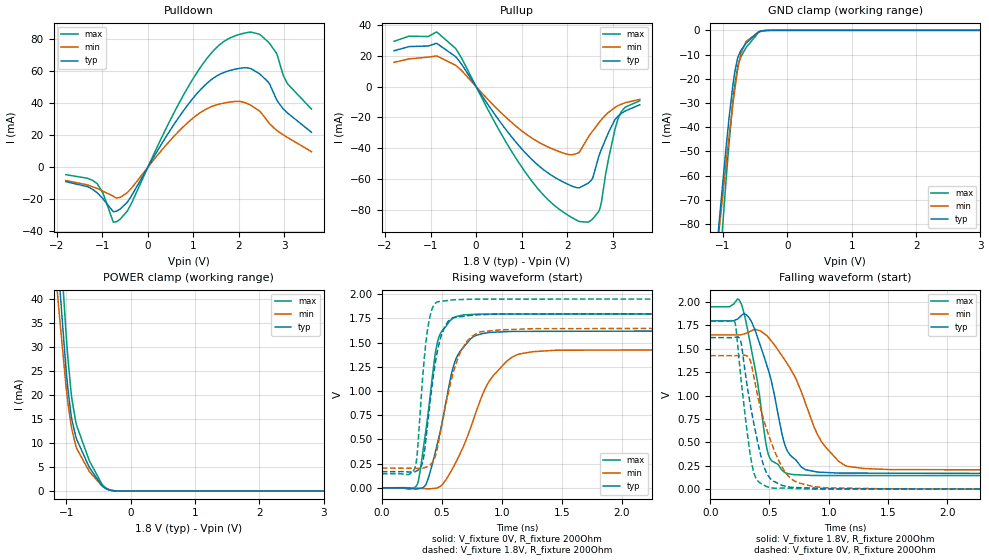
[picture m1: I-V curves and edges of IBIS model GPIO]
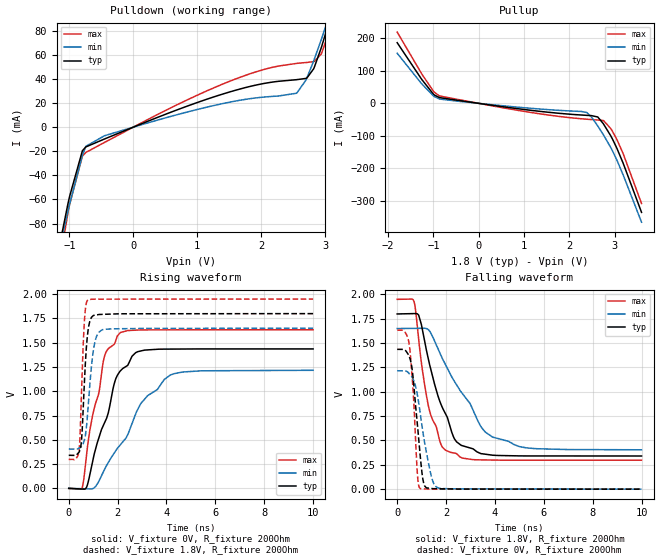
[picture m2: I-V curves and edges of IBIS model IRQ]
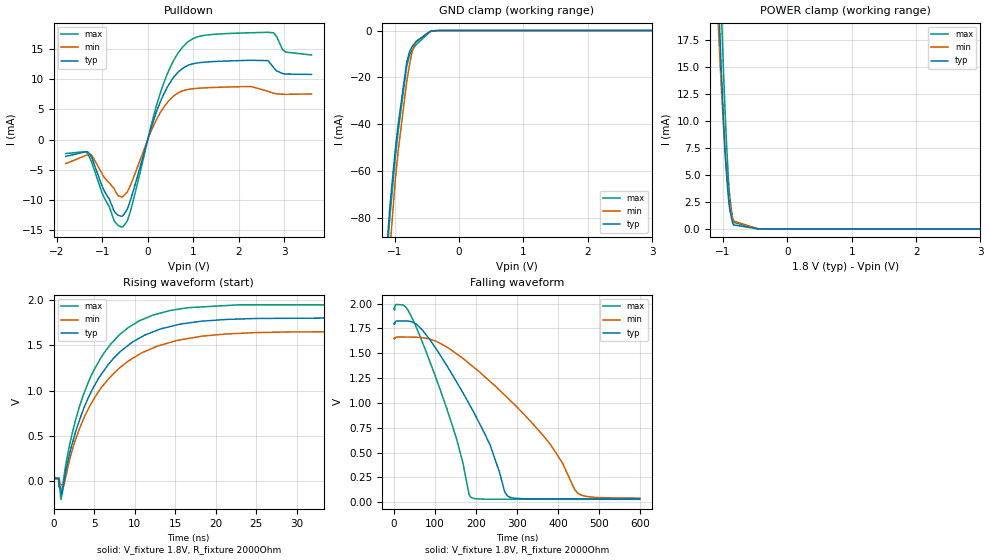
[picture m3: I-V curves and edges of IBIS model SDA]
|Texas Instruments Incorporated
| MIPI DSI Bridge To eDP
| Marketing part#   Digital Voltage Range   Package-type   #pins
| SN65DSI86   1.65V-1.95   PBGA   81
[IBIS Ver]   4.1
[File name]   sn65dsi86.ibs
[File Rev]   1.0
[Date]   09/19/2013
[Source]
| Texas Instruments Incorporated.
| Analog-eLab Design Center, HPA
| 12500 TI Blvd
| Dallas, TX -75243
| e-mail: elab_scm_ibis@list.ti.com
[Notes]   Revision History:
| Rev 1.0: 09/19/2013
| - Initial version of the model
| - Model generated from simulations in TISPICE
| - C_comp although listed in numerical order of value are
|   obtained from varying PVT conditions. For PVT conditions for
|   each specific value refer the buffer description under
|   respective [Model]. IBIS model user is responsible for using
|   appropriate C_comp to simulate for Signal Integrity.
| - Warnings regarding combined Non-monotonicity of various models have been
|   reviewd and considered minor and can be ignored.
| - DP output has sub models depending on the drive strength.
|   Please refer to the [Model Selector] section for details.
| - AUX pins has sub models depending on the drive strength.
|   Please refer to the [Model Selector] section for details.
[Disclaimer]
| This model is designed as an aid for customers of Texas Instruments.
| TI and its licensors and suppliers make no warranties, either expressed
| or implied, with respect to this  model, including the warranties of
| merchantability or fitness for a particular purpose. The model is
| provided solely on an "as is" basis. The entire risk as to its quality
| and performance is with the customer.
[Copyright]
 (C) Copyright 2013 Texas Instruments Incorporated.All rights reserved.
|   SN65DSI86
[Component]   SN65DSI86
[Manufacturer]   TI
[Package]
| variable   typ   min   max
R_pkg   0.1   0.08   0.12
L_pkg   0.7nH   0.56nH   0.84nH
C_pkg   0.1pF   0.08pF   0.12pF
[Pin]  signal_name   model_name   R_pin   L_pin   C_pin
A1   ADDR   input   NA   NA   NA
A2   VCCIO   POWER   NA   NA   NA
A3   IRQ   IRQ   NA   NA   NA
A4   GPIO1   GPIO   NA   NA   NA
A5   GPIO2   GPIO   NA   NA   NA
A6   GPIO3   GPIO   NA   NA   NA
A7   REFCLK   refclk_in   NA   NA   NA
A8   GND   GND   NA   NA   NA
A9   VCCA   POWER   NA   NA   NA
B1   EN   input_b   NA   NA   NA
B2   VCCA   POWER   NA   NA   NA
B3   TEST1   input_w_pd   NA   NA   NA
B4   GPIO4   GPIO   NA   NA   NA
B5   TEST2   input_w_pd   NA   NA   NA
B6   VCCIO   POWER   NA   NA   NA
B7   TEST3   input_w_pd   NA   NA   NA
B8   ML3P   DP_OUT   NA   NA   NA
B9   ML3N   DP_OUT   NA   NA   NA
C1   DB0N   DSI_INPUT   NA   NA   NA
C2   DB0P   DSI_INPUT   NA   NA   NA
C8   ML2P   DP_OUT   NA   NA   NA
C9   ML2N   DP_OUT   NA   NA   NA
D1   DB1N   DSI_INPUT   NA   NA   NA
D2   DB1P   DSI_INPUT   NA   NA   NA
D5   VCC   POWER   NA   NA   NA
D6   VCC   POWER   NA   NA   NA
D8   GND   GND   NA   NA   NA
D9   VPLL   POWER   NA   NA   NA
E1   DBCN   DSI_INPUT   NA   NA   NA
E2   DBCP   DSI_INPUT   NA   NA   NA
E4   GND   GND   NA   NA   NA
E5   GND   GND   NA   NA   NA
E6   VCCA   POWER   NA   NA   NA
E8   ML1P   DP_OUT   NA   NA   NA
E9   ML1N   DP_OUT   NA   NA   NA
F1   DB2N   DSI_INPUT   NA   NA   NA
F2   DB2P   DSI_INPUT   NA   NA   NA
F4   GND   GND   NA   NA   NA
F5   GND   GND   NA   NA   NA
F6   GND   GND   NA   NA   NA
F8   ML0P   DP_OUT   NA   NA   NA
F9   ML0N   DP_OUT   NA   NA   NA
G1   DB3N   DSI_INPUT   NA   NA   NA
G2   DB3P   DSI_INPUT   NA   NA   NA
G8   GND   GND   NA   NA   NA
G9   VCCA   POWER   NA   NA   NA
H1   SCL   SDA   NA   NA   NA
H2   VCCA   POWER   NA   NA   NA
H3   DA0P   LP_TX   NA   NA   NA
H4   DA1P   DSI_INPUT   NA   NA   NA
H5   DACP   DSI_INPUT   NA   NA   NA
H6   DA2P   DSI_INPUT   NA   NA   NA
H7   DA3P   DSI_INPUT   NA   NA   NA
H8   AUXP   AUX   NA   NA   NA
H9   AUXN   AUX   NA   NA   NA
J1   SDA   SDA   NA   NA   NA
J2   VCC   POWER   NA   NA   NA
J3   DA0N   LP_TX   NA   NA   NA
J4   DA1N   DSI_INPUT   NA   NA   NA
J5   DACN   DSI_INPUT   NA   NA   NA
J6   DA2N   DSI_INPUT   NA   NA   NA
J7   DA3N   DSI_INPUT   NA   NA   NA
J8   HPD   input_w_pd_b   NA   NA   NA
J9   VCC   POWER   NA   NA   NA
[Diff Pin]  inv_pin  vdiff  tdelay_typ tdelay_min tdelay_max
H3   J3   100mV   NA   NA   NA
H4   J4   100mV   NA   NA   NA
H6   J6   100mV   NA   NA   NA
H7   J7   100mV   NA   NA   NA
H5   J5   100mV   NA   NA   NA
C2   C1   100mV   NA   NA   NA
D2   D1   100mV   NA   NA   NA
F2   F1   100mV   NA   NA   NA
G2   G1   100mV   NA   NA   NA
E2   E1   100mV   NA   NA   NA
C8   C9   NA   NA   NA   NA
B8   B9   NA   NA   NA   NA
H8   H9   200mV   NA   NA   NA
E8   E9   NA   NA   NA   NA
F8   F9   NA   NA   NA   NA
|   Model Selectors
[Model Selector]  DP_OUT
DP_OUT_800   High swing DP output
DP_OUT_600   Medium swing DP output
DP_OUT_400   Low swing DP output
[Model Selector]  AUX
AUX_IO_1000   AUX output
AUX_IO_INPUT   AUX as an input buffer
[Model Selector]  LP_TX
LPTX_OUT   Buffer as an output
DSI_INPUT   Buffer as an input
| Models and submodels in the file (15): GPIO (I/O), IRQ (Output), SDA (I/O_open_drain), refclk_in (Input), LPTX_OUT (Output), input_w_pd_b (Input), input_w_pd (Input), input_b (Input), input (Input), DSI_INPUT (Input), DP_OUT_800 (Output), DP_OUT_600 (Output), DP_OUT_400 (Output), AUX_IO_INPUT (Input), AUX_IO_1000 (Output)
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|   Model
[Model]   GPIO
Model_type   I/O
Polarity   Non-Inverting
Enable   Active-Low
Vinl = 0.54
Vinh = 1.26
Vmeas = 0.9
Vref = 0
Cref = 1pF
Rref = 10000
|   typ   min   max
C_comp   0.4630pF   0.3789pF   0.6229pF
[Voltage Range]   1.8   1.65   1.95
[Temperature Range]   27   125   -40
[Pullup Reference]   1.8   1.65   1.95
[Pulldown Reference]   -0   -0   -0
[Power Clamp Reference]   1.8   1.65   1.95
[GND Clamp Reference]   -0   -0   -0
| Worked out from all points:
|   slope of the pulldown table from 0 to 0.27 V, typ, clamps not added: 20.6 ohm
|   slope of the pullup table from 0 to 0.27 V, typ, clamps not added: 22.3 ohm
|   GND clamp passes 1 mA (typ) near -0.46 V on its own axis
|   POWER clamp passes 1 mA (typ) near -0.44 V on its own axis
|   falling waveform, V_fixture 1.8V, R_fixture 200Ohm: 20-80 % time 186ps typ, 306ps min, 135ps max; typ from 1.8 V to 0.167 V
|   rising waveform, V_fixture 0V, R_fixture 200Ohm: 20-80 % time 170ps typ, 292ps min, 112ps max; typ from 0 V to 1.62 V
|   rising waveform, V_fixture 1.8V, R_fixture 200Ohm: 20-80 % time 107ps typ, 165ps min, 71.5ps max; typ from 0.167 V to 1.8 V
|   falling waveform, V_fixture 0V, R_fixture 200Ohm: 20-80 % time 145ps typ, 208ps min, 99.7ps max; typ from 1.62 V to 0 V
[Pulldown]
|   Voltage   I(typ)   I(min)   I(max)
-1.8V     -8.944mA   -8.235mA   -4.562mA
-1.114V   -15.8mA    -13.15mA   -10.13mA
-757.8mV  -27.74mA   -18.05mA   -34.18mA
-606.6mV  -26.07mA   -18.76mA   -32.41mA
-374.4mV  -18.55mA   -13.55mA   -23.38mA
1.062V    45.55mA    32.36mA    58.49mA
1.543V    57.62mA    39.35mA    75.79mA
2.045V    62.06mA    41.12mA    83.37mA
2.644V    53.32mA    28.38mA    78.42mA
2.822V    42.75mA    23.29mA    71.52mA
3.065V    34.07mA    18.73mA    52.33mA
3.595V    21.94mA    9.811mA    36.44mA
[GND Clamp]
|   Voltage   I(typ)   I(min)   I(max)
-1.8V     -365.9mA   -331.5mA   -431.2mA
-1.06V    -78.98mA   -82.24mA   -100.4mA
-952.2mV  -48.1mA    -54.78mA   -61.49mA
-903.6mV  -35.48mA   -43.14mA   -45.61mA
-849.6mV  -23.12mA   -31.03mA   -29.92mA
-817.2mV  -17.09mA   -24.36mA   -22.2mA
-774mV    -11.57mA   -16.51mA   -15.13mA
-720mV    -8.222mA   -9.272mA   -10.82mA
-639mV    -5.235mA   -4.533mA   -6.997mA
-450mV    -639.8uA   -729.1uA   -952.1uA
-266.4mV  -7.244uA   -17.61uA   -9.882uA
3.595V    0A         0A         0A
[Pullup]
|   Voltage   I(typ)   I(min)   I(max)
-1.8V     23.39mA    15.83mA    29.57mA
-860.4mV  28.1mA     19.91mA    35.51mA
-450mV    19.54mA    13.93mA    24.86mA
1.105V    -43.86mA   -31.05mA   -56.77mA
1.645V    -57.54mA   -40.13mA   -75.43mA
2.266V    -65.88mA   -42.69mA   -87.82mA
2.558V    -59.6mA    -28.9mA    -86.14mA
2.693V    -45.47mA   -23.7mA    -81.24mA
2.909V    -29.66mA   -16.65mA   -46.78mA
3.119V    -19.11mA   -12.37mA   -20.55mA
3.281V    -15.75mA   -10.4mA    -13.25mA
3.595V    -11.8mA    -8.235mA   -9.174mA
[POWER Clamp]
|   Voltage   I(typ)   I(min)   I(max)
-1.8V     199mA      166.7mA    232.1mA
-1.136V   48.46mA    40.77mA    60.31mA
-1.125V   46.37mA    39.03mA    57.88mA
-1.006V   25.5mA     21.9mA     33.07mA
-979.2mV  21.68mA    18.73mA    28.27mA
-919.8mV  15.28mA    13.2mA     19.79mA
-855mV    11.4mA     9.486mA    14.47mA
-639mV    4.811mA    3.978mA    6.176mA
-450mV    1.136mA    1.099mA    1.482mA
-390.6mV  522.3uA    551.4uA    697.5uA
-207mV    5.854uA    12.5uA     9.961uA
3.595V    0A         0A         0A
[Ramp]
R_load = 200
|   typ   min   max
dV/dt_r   0.972411/1.69676e-10   0.855528/2.91185e-10   1.07754/1.1156e-10
dV/dt_f   0.979876/1.85387e-10   0.866595/3.0597e-10   1.08306/1.34833e-10
[Falling Waveform]
V_fixture = 1.8V
V_fixture_min = 1.65V
V_fixture_max = 1.95V
R_fixture = 200Ohm
C_fixture = 0F
|   Time   V(typ)   V(min)   V(max)
0s        1.8V       1.649V     1.95V
258.4ps   1.851V     1.651V     1.992V
343.1ps   1.802V     1.69V      1.523V
395.3ps   1.638V     1.703V     1.174V
484.3ps   1.297V     1.632V     400.6mV
627.8ps   484.9mV    1.386V     179.8mV
767.4ps   239.1mV    1.047V     151.8mV
930.4ps   181.3mV    525.8mV    146.1mV
1.14ns    171.8mV    251.6mV    146mV
3ns       166.9mV    204.9mV    144.9mV
[Rising Waveform]
V_fixture = 0V
V_fixture_min = 0V
V_fixture_max = 0V
R_fixture = 200Ohm
C_fixture = 0F
|   Time   V(typ)   V(min)   V(max)
0s        21.86uV    715.5uV    748.1nV
296.3ps   -10.95mV   -3.704mV   37.73mV
371.1ps   44.67mV    -9.622mV   629.5mV
435.1ps   316.1mV    -5.576mV   1.293V
462.3ps   453.3mV    -2.002mV   1.499V
607.8ps   1.3V       242mV      1.763V
743.4ps   1.542V     632.4mV    1.79V
884.5ps   1.602V     1.08V      1.795V
1.127ns   1.616V     1.374V     1.795V
3ns       1.621V     1.427V     1.796V
[Rising Waveform]
V_fixture = 1.8V
V_fixture_min = 1.65V
V_fixture_max = 1.95V
R_fixture = 200Ohm
C_fixture = 0F
|   Time   V(typ)   V(min)   V(max)
0s        166.6mV    204.1mV    144.9mV
279ps     168mV      201.4mV    218.4mV
296.3ps   178.7mV    201.3mV    372.1mV
336.1ps   247.1mV    202.1mV    1.071V
375.4ps   588.6mV    216.9mV    1.585V
462.3ps   1.406V     408.5mV    1.92V
527.6ps   1.673V     825.8mV    1.932V
628.9ps   1.764V     1.321V     1.944V
808.6ps   1.788V     1.606V     1.95V
3ns       1.8V       1.648V     1.95V
[Falling Waveform]
|Gnd
V_fixture = 0V
V_fixture_min = 0V
V_fixture_max = 0V
R_fixture = 200Ohm
C_fixture = 0F
|   Time   V(typ)   V(min)   V(max)
0s        1.621V     1.428V     1.796V
209.8ps   1.624V     1.427V     1.782V
262.3ps   1.557V     1.43V      1.152V
315.3ps   1.079V     1.422V     580.1mV
354.1ps   794.2mV    1.293V     252.3mV
395.3ps   535mV      1.028V     98.12mV
474.3ps   178.2mV    647.9mV    28.27mV
643.5ps   29.61mV    163mV      11mV
870ps     11.51mV    27.93mV    1.006mV
3ns       234.7uV    1.411mV    1.146uV
|   Model
[Model]   IRQ
Model_type   Output
Polarity   Non-Inverting
Vmeas = 0.9
Vref = 0
Cref = 1pF
Rref = 10000
|   typ   min   max
C_comp   0.2695pF   0.2096pF   0.3469pF
[Voltage Range]   1.8   1.65   1.95
[Temperature Range]   27   125   -40
[Pullup Reference]   1.8   1.65   1.95
[Pulldown Reference]   -0   -0   -0
[Power Clamp Reference]   1.8   1.65   1.95
[GND Clamp Reference]   -0   -0   -0
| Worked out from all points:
|   slope of the pulldown table from 0 to 0.27 V, typ, clamps not added: 46.5 ohm
|   slope of the pullup table from 0 to 0.27 V, typ, clamps not added: 50.4 ohm
|   falling waveform, V_fixture 1.8V, R_fixture 200Ohm: 20-80 % time 1.04ns typ, 1.66ns min, 767ps max; typ from 1.8 V to 0.341 V
|   rising waveform, V_fixture 0V, R_fixture 200Ohm: 20-80 % time 974ps typ, 1.78ns min, 693ps max; typ from 0 V to 1.44 V
|   rising waveform, V_fixture 1.8V, R_fixture 200Ohm: 20-80 % time 183ps typ, 265ps min, 143ps max; typ from 0.341 V to 1.8 V
|   falling waveform, V_fixture 0V, R_fixture 200Ohm: 20-80 % time 314ps typ, 477ps min, 223ps max; typ from 1.44 V to 0 V
[Pulldown]
|   Voltage   I(typ)   I(min)   I(max)
-1.8V     -333mA     -309.7mA   -367.4mA
-1.157V   -99.32mA   -101.7mA   -114.1mA
-1.022V   -63.77mA   -69.97mA   -71.37mA
-795.6mV  -19.54mA   -23.42mA   -24.05mA
-741.6mV  -16.41mA   -15.88mA   -20.97mA
1.289V    25.61mA    18.28mA    33.3mA
2.552V    39.37mA    28.13mA    52.87mA
2.817V    48.31mA    54.73mA    54.33mA
2.936V    65.68mA    72.46mA    60.58mA
3.022V    80.75mA    86.06mA    73.32mA
3.071V    89.66mA    93.88mA    82.17mA
3.595V    192.5mA    182mA      195.1mA
[Pullup]
|   Voltage   I(typ)   I(min)   I(max)
-1.8V     186.6mA    154.1mA    219.3mA
-1.249V   72.09mA    58.72mA    88.81mA
-1.001V   28.48mA    23.16mA    37.43mA
-871.2mV  17.99mA    13.71mA    23.36mA
1.062V    -19.91mA   -14.15mA   -26mA
2.385V    -36.91mA   -28.19mA   -48.82mA
2.628V    -41.93mA   -69.51mA   -51.27mA
2.758V    -64.03mA   -97.92mA   -53.23mA
2.914V    -99.8mA    -135.6mA   -77.48mA
3.049V    -137.9mA   -174.4mA   -111mA
3.19V     -184.6mA   -220.4mA   -155.2mA
3.595V    -335.4mA   -365.7mA   -308.2mA
[Ramp]
R_load = 200
|   typ   min   max
dV/dt_r   0.861892/9.76011e-10   0.729729/1.75843e-09   0.980234/6.94517e-10
dV/dt_f   0.875592/1.04381e-09   0.74723/1.6614e-09   0.991498/7.69733e-10
[Falling Waveform]
V_fixture = 1.8V
V_fixture_min = 1.65V
V_fixture_max = 1.95V
R_fixture = 200Ohm
C_fixture = 0F
|   Time   V(typ)   V(min)   V(max)
0s        1.8V       1.65V      1.95V
688.8ps   1.804V     1.652V     1.929V
878.6ps   1.788V     1.652V     1.542V
1.269ns   1.345V     1.639V     866.8mV
1.98ns    773.2mV    1.278V     400.9mV
2.433ns   485.8mV    1.071V     363.2mV
3.452ns   364.5mV    633mV      300.9mV
3.913ns   348.7mV    535.4mV    299.1mV
5.421ns   341.3mV    420.9mV    297.5mV
10ns      340.7mV    404.5mV    297.5mV
[Rising Waveform]
V_fixture = 0V
V_fixture_min = 0V
V_fixture_max = 0V
R_fixture = 200Ohm
C_fixture = 0F
|   Time   V(typ)   V(min)   V(max)
0s        62.16nV    120uV      254.8nV
556.8ps   -7.315mV   -3.762mV   8.38mV
864.8ps   142.5mV    -5.909mV   600mV
1.244ns   529.9mV    79.93mV    998.9mV
1.455ns   669.9mV    189mV      1.353V
1.873ns   1.089V     368.3mV    1.489V
2.103ns   1.208V     446.3mV    1.603V
2.964ns   1.416V     878.1mV    1.632V
4.245ns   1.435V     1.176V     1.633V
10ns      1.436V     1.216V     1.634V
[Rising Waveform]
V_fixture = 1.8V
V_fixture_min = 1.65V
V_fixture_max = 1.95V
R_fixture = 200Ohm
C_fixture = 0F
|   Time   V(typ)   V(min)   V(max)
0s        340.7mV    404.5mV    297.5mV
420ps     373.3mV    413.6mV    387.1mV
461.5ps   396.6mV    418.6mV    540.7mV
524ps     500.2mV    435.1mV    996.3mV
636.5ps   1.069V     496.6mV    1.705V
710.1ps   1.41V      602.3mV    1.896V
788.7ps   1.623V     825.1mV    1.942V
1.031ns   1.782V     1.456V     1.948V
1.347ns   1.792V     1.631V     1.949V
10ns      1.8V       1.65V      1.95V
[Falling Waveform]
|Gnd
V_fixture = 0V
V_fixture_min = 0V
V_fixture_max = 0V
R_fixture = 200Ohm
C_fixture = 0F
|   Time   V(typ)   V(min)   V(max)
0s        1.436V     1.216V     1.634V
311.8ps   1.428V     1.216V     1.615V
496.9ps   1.361V     1.185V     1.481V
654.9ps   1.137V     1.127V     1.001V
831.4ps   651.9mV    961.3mV    141.8mV
942.1ps   345mV      780.9mV    7.068mV
1.127ns   32.18mV    470.2mV    3.116mV
1.45ns    5.693mV    88.88mV    790.7uV
1.674ns   4.342mV    12.77mV    770uV
10ns      62.02nV    120.2uV    254.7nV
|   Model
[Model]   SDA
Model_type   I/O_open_drain
Polarity   Non-Inverting
Enable   Active-Low
Vinl = 0.54
Vinh = 1.26
Vmeas = 0.9
Vref = 1.8
Cref = 1pF
Rref = 2000
|   typ   min   max
C_comp   0.4063pF   0.3201pF   0.4932pF
[Voltage Range]   1.8   1.65   1.95
[Temperature Range]   27   125   -40
[Pullup Reference]   1.8   1.65   1.95
[Pulldown Reference]   -0   -0   -0
[Power Clamp Reference]   1.8   1.65   1.95
[GND Clamp Reference]   -0   -0   -0
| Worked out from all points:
|   slope of the pulldown table from 0 to 0.27 V, typ, clamps not added: 44.3 ohm
|   GND clamp passes 1 mA (typ) near -0.48 V on its own axis
|   POWER clamp passes 1 mA (typ) near -0.87 V on its own axis
|   falling waveform, V_fixture 1.8V, R_fixture 2000Ohm: 20-80 % time 133ns typ, 211ns min, 93.5ns max; typ from 1.8 V to 0.033 V
|   rising waveform, V_fixture 1.8V, R_fixture 2000Ohm: 20-80 % time 6.22ns typ, 6.88ns min, 5.6ns max; typ from 0.033 V to 1.8 V
[Pulldown]
|   Voltage   I(typ)   I(min)   I(max)
-1.8V     -2.775mA   -3.966mA   -2.31mA
-1.357V   -2.016mA   -2.616mA   -1.971mA
-1.228V   -3.037mA   -2.635mA   -3.85mA
-741.6mV  -11.77mA   -8.078mA   -13.35mA
-547.2mV  -12.58mA   -9.429mA   -14.42mA
-374.4mV  -9.845mA   -7.437mA   -11.63mA
306mV     6.753mA    4.837mA    8.369mA
835.2mV   12.07mA    8.193mA    15.8mA
2.266V    13.08mA    8.754mA    17.62mA
2.758V    11.94mA    7.639mA    17.62mA
3.028V    10.8mA     7.46mA     14.43mA
3.595V    10.74mA    7.52mA     13.95mA
[GND Clamp]
|   Voltage   I(typ)   I(min)   I(max)
-1.8V     -584.9mA   -593.4mA   -587.7mA
-1.114V   -89.8mA    -112.3mA   -93.69mA
-1.082V   -77.55mA   -96.92mA   -81.84mA
-1.071V   -73.87mA   -92.25mA   -78.17mA
-995.4mV  -52.02mA   -65.11mA   -55.54mA
-946.8mV  -40.11mA   -51.48mA   -43.05mA
-806.4mV  -12.73mA   -20.71mA   -14.42mA
-768.6mV  -8.918mA   -14.34mA   -10.5mA
-725.4mV  -6.688mA   -8.715mA   -8.197mA
-666mV    -4.741mA   -4.563mA   -5.991mA
-450mV    -340.3uA   -406.7uA   -515.3uA
3.595V    0A         0A         0A
[POWER Clamp]
|   Voltage   I(typ)   I(min)   I(max)
-1.8V     160.5mA    134.1mA    187.1mA
-1.071V   21.35mA    18.46mA    28.34mA
-1.066V   20.49mA    17.78mA    27.33mA
-1.033V   15.58mA    13.84mA    21.4mA
-1.012V   12.54mA    11.4mA     17.66mA
-963mV    6.674mA    6.674mA    10.11mA
-919.8mV  3.033mA    3.571mA    4.947mA
-898.2mV  1.861mA    2.46mA     3.113mA
-855mV    598.6uA    1.047mA    989.3uA
-838.8mV  377.2uA    737.7uA    607uA
-450mV    369.4pA    86.94nA    24.51nA
3.595V    0A         0A         0A
[Ramp]
R_load = 2000
|   typ   min   max
dV/dt_r   1.06013/6.22272e-09   0.965093/6.88395e-09   1.15222/5.59552e-09
dV/dt_f   1.06013/1.32582e-07   0.964806/2.11092e-07   1.15222/9.34972e-08
[Falling Waveform]
V_fixture = 1.8V
V_fixture_min = 1.65V
V_fixture_max = 1.95V
R_fixture = 2000Ohm
C_fixture = 0F
|   Time   V(typ)   V(min)   V(max)
0s        1.8V       1.65V      1.95V
26.88ns   1.825V     1.662V     1.97V
60.63ns   1.767V     1.66V      1.697V
142.7ns   1.278V     1.522V     764.8mV
186.7ns   963.8mV    1.385V     53.22mV
234.9ns   570.1mV    1.213V     30.47mV
281.5ns   52.05mV    1.032V     30.32mV
381.2ns   34.76mV    584.5mV    30.01mV
449.1ns   33.82mV    89.43mV    29.79mV
600ns     33.11mV    41.95mV    29.63mV
[Rising Waveform]
V_fixture = 1.8V
V_fixture_min = 1.65V
V_fixture_max = 1.95V
R_fixture = 2000Ohm
C_fixture = 0F
|   Time   V(typ)   V(min)   V(max)
0s        33.11mV    41.47mV    29.63mV
622.9ps   33.58mV    41.88mV    30.53mV
915.9ps   -92.68mV   -32.79mV   -196.7mV
1.256ns   -28.93mV   -48.18mV   33.93mV
2.052ns   329.9mV    262.4mV    431.7mV
3.668ns   791.6mV    681.4mV    949.1mV
8.147ns   1.422V     1.251V     1.617V
13.29ns   1.683V     1.504V     1.858V
22.75ns   1.789V     1.631V     1.946V
600ns     1.8V       1.65V      1.95V
